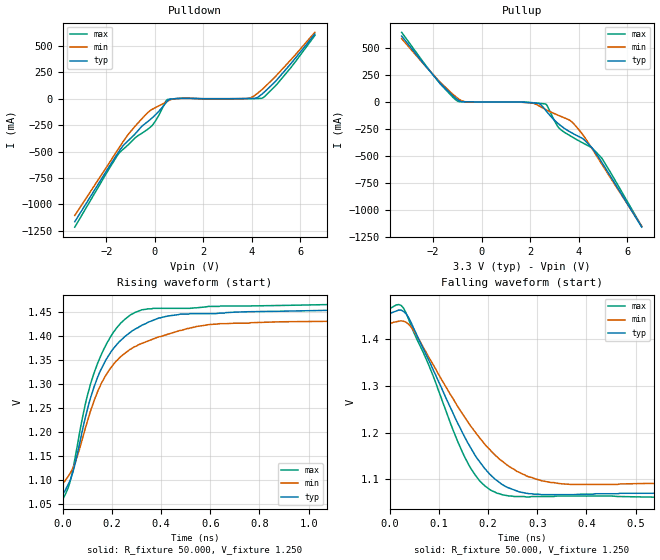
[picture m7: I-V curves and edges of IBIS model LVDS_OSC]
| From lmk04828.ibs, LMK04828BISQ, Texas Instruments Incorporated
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|   Model LVDS
[Model]   LVDS_OSC
Model_type   Output
Polarity   Non-Inverting
Vmeas = 1.25
Vref = 1.25
Cref = 0pF
Rref = 50
|   typ   min   max
|   (nom PVT)   (slow PVT)   (fast PVT)
C_comp   1.2694p   1.2464p   1.3920p
|C_comp (High state)   1.2694p   1.2464p   1.3920p
|C_comp (Low state)   1.7368p   1.7367p   1.7369p
[Voltage Range]   3.3   3.15   3.45
[Temperature Range]   27   125   -40
[Pullup Reference]   3.3   3.15   3.45
[Pulldown Reference]   0   0   -0
[Power Clamp Reference]   3.3   3.15   3.45
[GND Clamp Reference]   0   0   0
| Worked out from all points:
|   slope of the pulldown table from 0 to 0.495 V, typ, clamps not added: 3.84 ohm
|   slope of the pullup table from 0 to 0.495 V, typ, clamps not added: 3.12 kohm
|   falling waveform, R_fixture 50.000, V_fixture 1.250: 20-80 % time 107ps typ, 127ps min, 93.2ps max; typ from 1.46 V to 1.07 V
|   rising waveform, R_fixture 50.000, V_fixture 1.250: 20-80 % time 156ps typ, 191ps min, 131ps max; typ from 1.07 V to 1.46 V
[Pulldown]
|   Voltage   I(typ)   I(min)   I(max)
-3.3V     -1.164A    -1.105A    -1.215A
-1.556V   -525.8mA   -492.8mA   -540.2mA
-1.078V   -393.2mA   -332mA     -432.4mA
-395.3mV  -235mA     -155.4mA   -305.6mA
-84.48mV  -175.9mA   -97.08mA   -246.8mA
521.4mV   -21.65mA   -23.87mA   -7.381mA
1.092V    3.707mA    3.082mA    4.094mA
3.814V    1.636mA    2.314mA    1.277mA
4.133V    3.419mA    33.61mA    1.998mA
4.41V     42.13mA    85.11mA    4.134mA
5.01V     173.2mA    219.4mA    130.8mA
6.598V    611.4mA    628.3mA    598.5mA
[Pullup]
|   Voltage   I(typ)   I(min)   I(max)
-3.3V     611.6mA    587.6mA    646.1mA
-1.712V   173.7mA    183.8mA    169mA
-965.6mV  16.51mA    30.77mA    4.506mA
-684.4mV  1.966mA    2.606mA    2.029mA
2.27V     -11.76mA   -24.81mA   -10.16mA
2.628V    -74.37mA   -68.56mA   -18.92mA
3.19V     -207mA     -126.8mA   -242.4mA
3.674V    -281.4mA   -176.2mA   -316.8mA
4.256V    -356.4mA   -330.7mA   -390.2mA
4.541V    -424mA     -429.7mA   -426.3mA
4.955V    -560.3mA   -577.4mA   -522.1mA
6.598V    -1.161A    -1.153A    -1.154A
[Ramp]
R_load = 50
|   typ   min   max
dV/dt_r   0.230311/1.56545e-10   0.20357/1.9031e-10   0.24665/1.30209e-10
dV/dt_f   0.230311/1.07194e-10   0.20357/1.26958e-10   0.24665/9.33894e-11
[Falling Waveform]
R_fixture = 50.000
V_fixture = 1.250
V_fixture_min = 1.250
V_fixture_max = 1.250
C_fixture = 0.000
|  time   V(typ)   V(min)   V(max)
|   0.000S   1.455V   1.434V   1.466V
|   90.000pS   1.455V   1.434V   1.466V
|   95.000pS   1.455V   1.434V   1.466V
|  100.000pS   1.455V   1.434V   1.466V
|  105.000pS   1.456V   1.435V   1.467V
|  110.000pS   1.457V   1.435V   1.468V
|  115.000pS   1.459V   1.437V   1.471V
|  120.000pS   1.461V   1.438V   1.474V
|  125.000pS   1.463V   1.439V   1.475V
|  130.000pS   1.463V   1.440V   1.473V
|  135.000pS   1.460V   1.439V   1.467V
|  140.000pS   1.455V   1.437V   1.457V
|  145.000pS   1.447V   1.433V   1.444V
|  150.000pS   1.437V   1.427V   1.430V
|  155.000pS   1.425V   1.420V   1.417V
|  160.000pS   1.414V   1.412V   1.405V
|  165.000pS   1.402V   1.402V   1.394V
|  170.000pS   1.391V   1.393V   1.383V
|  175.000pS   1.380V   1.383V   1.372V
|  180.000pS   1.369V   1.374V   1.360V
|  185.000pS   1.358V   1.364V   1.348V
|  190.000pS   1.347V   1.355V   1.335V
|  195.000pS   1.335V   1.346V   1.322V
|  200.000pS   1.324V   1.337V   1.308V
|  205.000pS   1.312V   1.327V   1.293V
|  210.000pS   1.301V   1.318V   1.279V
|  215.000pS   1.289V   1.309V   1.264V
|  220.000pS   1.277V   1.300V   1.250V
|  230.000pS   1.254V   1.282V   1.221V
|  235.000pS   1.243V   1.274V   1.207V
|  240.000pS   1.231V   1.265V   1.194V
|  245.000pS   1.220V   1.256V   1.181V
|  250.000pS   1.210V   1.248V   1.169V
|  255.000pS   1.199V   1.240V   1.157V
|  260.000pS   1.189V   1.232V   1.146V
|  265.000pS   1.179V   1.224V   1.136V
|  270.000pS   1.170V   1.216V   1.126V
|  275.000pS   1.161V   1.209V   1.118V
|  280.000pS   1.152V   1.202V   1.110V
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0s        1.455V     1.434V     1.466V
18.33ps   1.463V     1.439V     1.475V
33.33ps   1.455V     1.437V     1.457V
53.33ps   1.414V     1.412V     1.405V
163.3ps   1.17V      1.216V     1.126V
193.3ps   1.123V     1.175V     1.086V
228.3ps   1.089V     1.139V     1.067V
283.3ps   1.069V     1.105V     1.062V
368.3ps   1.067V     1.089V     1.064V
1.883ns   1.071V     1.095V     1.06V
[Rising Waveform]
R_fixture = 50.000
V_fixture = 1.250
V_fixture_min = 1.250
V_fixture_max = 1.250
C_fixture = 0.000
|  time   V(typ)   V(min)   V(max)
|   0.000S   1.071V   1.095V   1.060V
|  105.000pS   1.071V   1.095V   1.059V
|  110.000pS   1.073V   1.095V   1.062V
|  115.000pS   1.076V   1.097V   1.067V
|  120.000pS   1.081V   1.101V   1.072V
|  125.000pS   1.086V   1.104V   1.078V
|  130.000pS   1.091V   1.108V   1.084V
|  135.000pS   1.096V   1.112V   1.092V
|  140.000pS   1.102V   1.116V   1.101V
|  145.000pS   1.110V   1.121V   1.112V
|  150.000pS   1.118V   1.126V   1.124V
|  155.000pS   1.128V   1.132V   1.138V
|  160.000pS   1.138V   1.139V   1.152V
|  165.000pS   1.150V   1.147V   1.166V
|  170.000pS   1.161V   1.155V   1.180V
|  175.000pS   1.173V   1.163V   1.195V
|  180.000pS   1.185V   1.172V   1.209V
|  185.000pS   1.197V   1.181V   1.222V
|  190.000pS   1.209V   1.190V   1.235V
|  195.000pS   1.220V   1.199V   1.247V
|  200.000pS   1.231V   1.209V   1.259V
|  205.000pS   1.241V   1.217V   1.270V
|  210.000pS   1.251V   1.226V   1.280V
|  215.000pS   1.261V   1.234V   1.289V
|  220.000pS   1.270V   1.243V   1.299V
|  225.000pS   1.278V   1.250V   1.307V
|  230.000pS   1.287V   1.258V   1.315V
|  235.000pS   1.294V   1.265V   1.323V
|  240.000pS   1.301V   1.272V   1.330V
|  245.000pS   1.308V   1.278V   1.337V
|  250.000pS   1.315V   1.285V   1.344V
|  255.000pS   1.321V   1.291V   1.350V
|  260.000pS   1.327V   1.296V   1.356V
|  265.000pS   1.332V   1.302V   1.362V
|  275.000pS   1.342V   1.311V   1.373V
|  280.000pS   1.347V   1.316V   1.378V
|  285.000pS   1.352V   1.320V   1.383V
|  290.000pS   1.356V   1.324V   1.388V
|  295.000pS   1.360V   1.328V   1.392V
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0s        1.071V     1.095V     1.06V
27ps      1.096V     1.112V     1.092V
47ps      1.128V     1.132V     1.138V
97ps      1.241V     1.217V     1.27V
142ps     1.315V     1.285V     1.344V
207ps     1.375V     1.342V     1.409V
292ps     1.414V     1.378V     1.449V
427ps     1.442V     1.404V     1.458V
637ps     1.448V     1.426V     1.462V
1.882ns   1.455V     1.434V     1.466V
